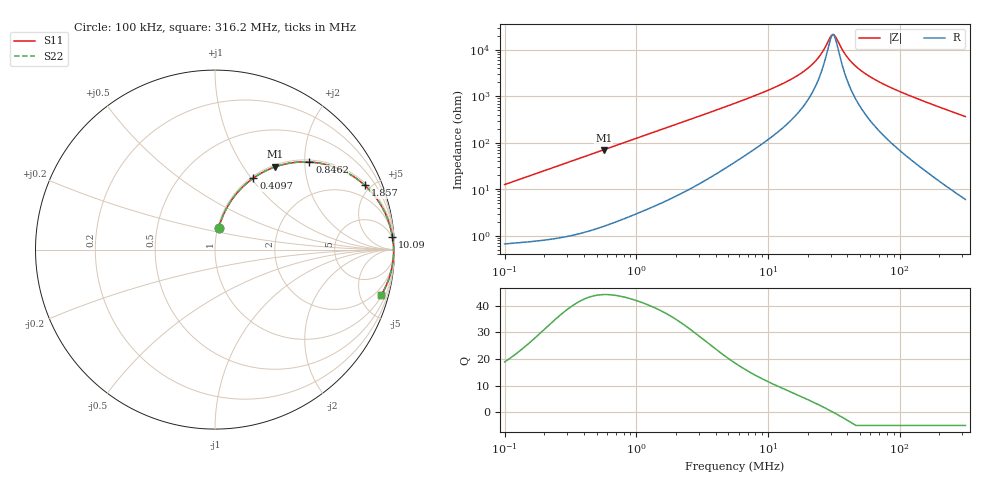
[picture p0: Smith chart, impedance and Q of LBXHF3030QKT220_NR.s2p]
! LBXHF3030QKT220_NR  S-PARAMETER MODEL  ( General Type )
! Model Generated by TAIYO YUDEN Corporation (http://www.ty-top.com)
! Version 1.0
! TAIYO YUDEN Control No. 210113NI43SB-FBB
! Copyright(c) 2021 TAIYO YUDEN CO.,LTD. All Rights Reserved.
! Product Description (link to TY-COMPAS)
! https://ds.yuden.co.jp/TYCOMPAS/or/detail?pn=LBXHF3030QKT220MNR&u=M
! Products Name : Inductors
! Characteristics :
!  Inductance : 22 uH , SRF(min) : 10 MHz , DC Resistance(max) : 0.504 Ohm
!  Rated Current : Saturation :510 mA , Temp Rise : 530 mA
!  Case Size : 3.0 x 3.0 / 0.118 x 0.118 [mm/inch] , Thickness : 1.5 / 0.059 [mm/inch]
!  (Conditions: Temperature = 25 degC , DC Bias Current/Voltage = 0A / 0V)
! External Node Assignments :
!  1  o---GGG---o  2
! GND o---------o GND
! Frequency Range : 0.1MHz  -  316.199832MHz  [ 402 STEP ]
# MHz S RI R 50
! Freq[MHz].  S11 Real  S11 Imag  S21 Real  S21 Imag  S12 Real  S12 Imag  S22 Real  S22 Imag
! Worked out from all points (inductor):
!   401 points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, 100 kHz to 316.2 MHz, reference 50 ohm
!   read as one part in series: L = 20.1 uH near 104.1 kHz
!   highest Q = 44.1 at 565.6 kHz (marker M1), where L = 19.9 uH
!   self-resonance near 31.17 MHz
!   S11 on the Smith chart (normalised r, x): 100 kHz: 1.01, +0.25; 409.7 kHz: 1.02, +1.03; 846.2 kHz: 1.05, +2.11; 1.857 MHz: 1.13, +4.61; 10.09 MHz: 3, +27; 316.2 MHz: 1.12, -7.33
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0.1  0.0221 0.1229  0.9779 -0.1229  0.9779 -0.1229  0.0221 0.1229
0.215029  0.0747 0.248  0.9253 -0.248  0.9253 -0.248  0.0747 0.248
0.385695  0.1951 0.3845  0.8049 -0.3845  0.8049 -0.3845  0.1951 0.3845
0.409726  0.214 0.3986  0.786 -0.3986  0.786 -0.3986  0.214 0.3986
0.565577  0.3369 0.4614  0.6631 -0.4614  0.6631 -0.4614  0.3369 0.4614
0.846233  0.5261 0.4878  0.4739 -0.4878  0.4739 -0.4878  0.5261 0.4878
1.487603  0.7675 0.4096  0.2325 -0.4096  0.2325 -0.4096  0.7675 0.4096
1.856676  0.8346 0.3578  0.1654 -0.3578  0.1654 -0.3578  0.8346 0.3578
3.01116  0.9259 0.245  0.0741 -0.245  0.0741 -0.245  0.9259 0.245
5.623165  0.9735 0.1358  0.0265 -0.1358  0.0265 -0.1358  0.9735 0.1358
10.08621  0.9884 0.072  0.0116 -0.072  0.0116 -0.072  0.9884 0.072
16.03156  0.993 0.0378  0.00696 -0.0378  0.00696 -0.0378  0.993 0.0378
21.68824  0.9946 0.0198  0.00545 -0.0198  0.00545 -0.0198  0.9946 0.0198
25.48142  0.995 0.0109  0.00498 -0.0109  0.00498 -0.0109  0.995 0.0109
29.93801  0.9953 0.00222  0.0047 -0.00222  0.0047 -0.00222  0.9953 0.00222
31.80333  0.9954 -0.00102  0.00465 0.00102  0.00465 0.00102  0.9954 -0.00102
38.90197  0.9954 -0.0119  0.00465 0.0119  0.00465 0.0119  0.9954 -0.0119
45.70575  0.9951 -0.021  0.00486 0.021  0.00486 0.021  0.9951 -0.021
59.39086  0.9943 -0.037  0.00571 0.037  0.00571 0.037  0.9943 -0.037
83.65039  0.9919 -0.0619  0.00813 0.0619  0.00813 0.0619  0.9919 -0.0619
153.0964  0.9799 -0.1246  0.0201 0.1246  0.0201 0.1246  0.9799 -0.1246
316.1998  0.9272 -0.2517  0.0728 0.2517  0.0728 0.2517  0.9272 -0.2517
